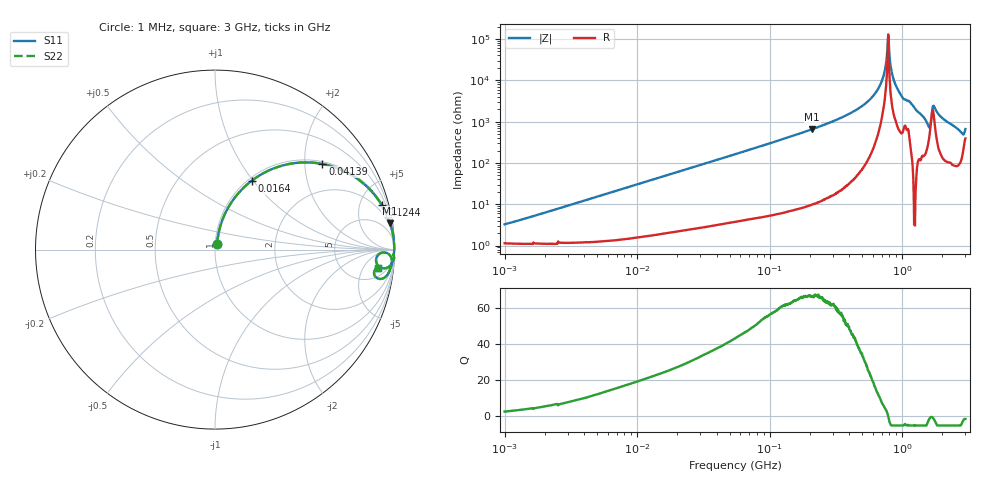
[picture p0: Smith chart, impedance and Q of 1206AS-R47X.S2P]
!s-Parameter Generated by FASTRON Sdn. Bhd.
!FASTRON P/N : 1206AS-R47X
!Keysight Technologies: E4991B_MY54100416_A.01.15
!Date created: Thu Nov 16 13:07:22 2023
!Version  : Rev00 Thu Nov 16 13:07:22 2023
!Data & Calibration Information:
!Freq	S11	S21	S12	S22
!PortZ  Port1:50+j0  Port2:50+j0
!When reading reference impedance value at option line is always used.
! Remarks : This data is being provided solely for informational purposes.
# Hz S dB R 50
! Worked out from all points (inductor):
!   1601 points, 1 MHz to 3 GHz, reference 50 ohm
!   read as one part in series: L = 487 nH near 1.094 MHz
!   highest Q = 66.9 at 209.4 MHz (marker M1), where L = 498 nH
!   self-resonance near 784.7 MHz
!   S11 on the Smith chart (normalised r, x): 1 MHz: 1.02, +0.06; 16.4 MHz: 1.04, +0.98; 41.39 MHz: 1.06, +2.45; 124.4 MHz: 1.12, +7.46; 3 GHz: 9, -11
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1000000  -29.82 67.9  -0.10 -1.7  -0.10 -1.7  -29.82 67.9
3804036  -18.83 77.6  -0.16 -6.5  -0.16 -6.5  -18.83 77.6
1.447069e7  -8.12 64.5  -0.89 -23.1  -0.89 -23.1  -8.12 64.5
1.639907e7  -7.24 62.0  -1.08 -25.7  -1.08 -25.7  -7.24 62.0
4.138676e7  -2.32 38.6  -4.10 -49.9  -4.10 -49.9  -2.32 38.6
5.477226e7  -1.49 31.3  -5.69 -57.4  -5.69 -57.4  -1.49 31.3
1.244416e8  -0.34 14.9  -11.77 -74.1  -11.77 -74.1  -0.34 14.9
2.083556e8  -0.12 8.7  -16.41 -80.4  -16.41 -80.4  -0.12 8.7
2.094008e8  -0.12 8.6  -16.46 -80.5  -16.46 -80.5  -0.12 8.6
3.933705e8  -0.03 3.8  -23.63 -85.1  -23.63 -85.1  -0.03 3.8
5.696638e8  -0.01 1.7  -30.70 -85.9  -30.70 -85.9  -0.01 1.7
6.924261e8  -0.01 0.7  -38.74 -82.9  -38.74 -82.9  -0.01 0.7
7.316083e8  -0.01 0.4  -43.40 -79.0  -43.40 -79.0  -0.01 0.4
7.653101e8  -0.01 0.1  -51.22 -69.5  -51.22 -69.5  -0.01 0.1
7.925923e8  -0.01 -0.1  -58.11 54.2  -58.11 54.2  -0.01 -0.1
8.543737e8  -0.01 -0.5  -41.24 80.6  -41.24 80.6  -0.01 -0.5
9.490412e8  -0.02 -1.1  -34.36 82.1  -34.36 82.1  -0.02 -1.1
1.565327e9  -0.38 -6.2  -18.85 64.9  -18.85 64.9  -0.38 -6.2
1.747494e9  -0.18 -2.2  -27.37 60.1  -27.37 60.1  -0.18 -2.2
2.000286e9  -0.11 -4.6  -21.93 79.0  -21.93 79.0  -0.11 -4.6
2.783064e9  -0.45 -9.7  -15.26 68.4  -15.26 68.4  -0.45 -9.7
3e9  -0.80 -6.4  -17.22 47.3  -17.22 47.3  -0.80 -6.4
